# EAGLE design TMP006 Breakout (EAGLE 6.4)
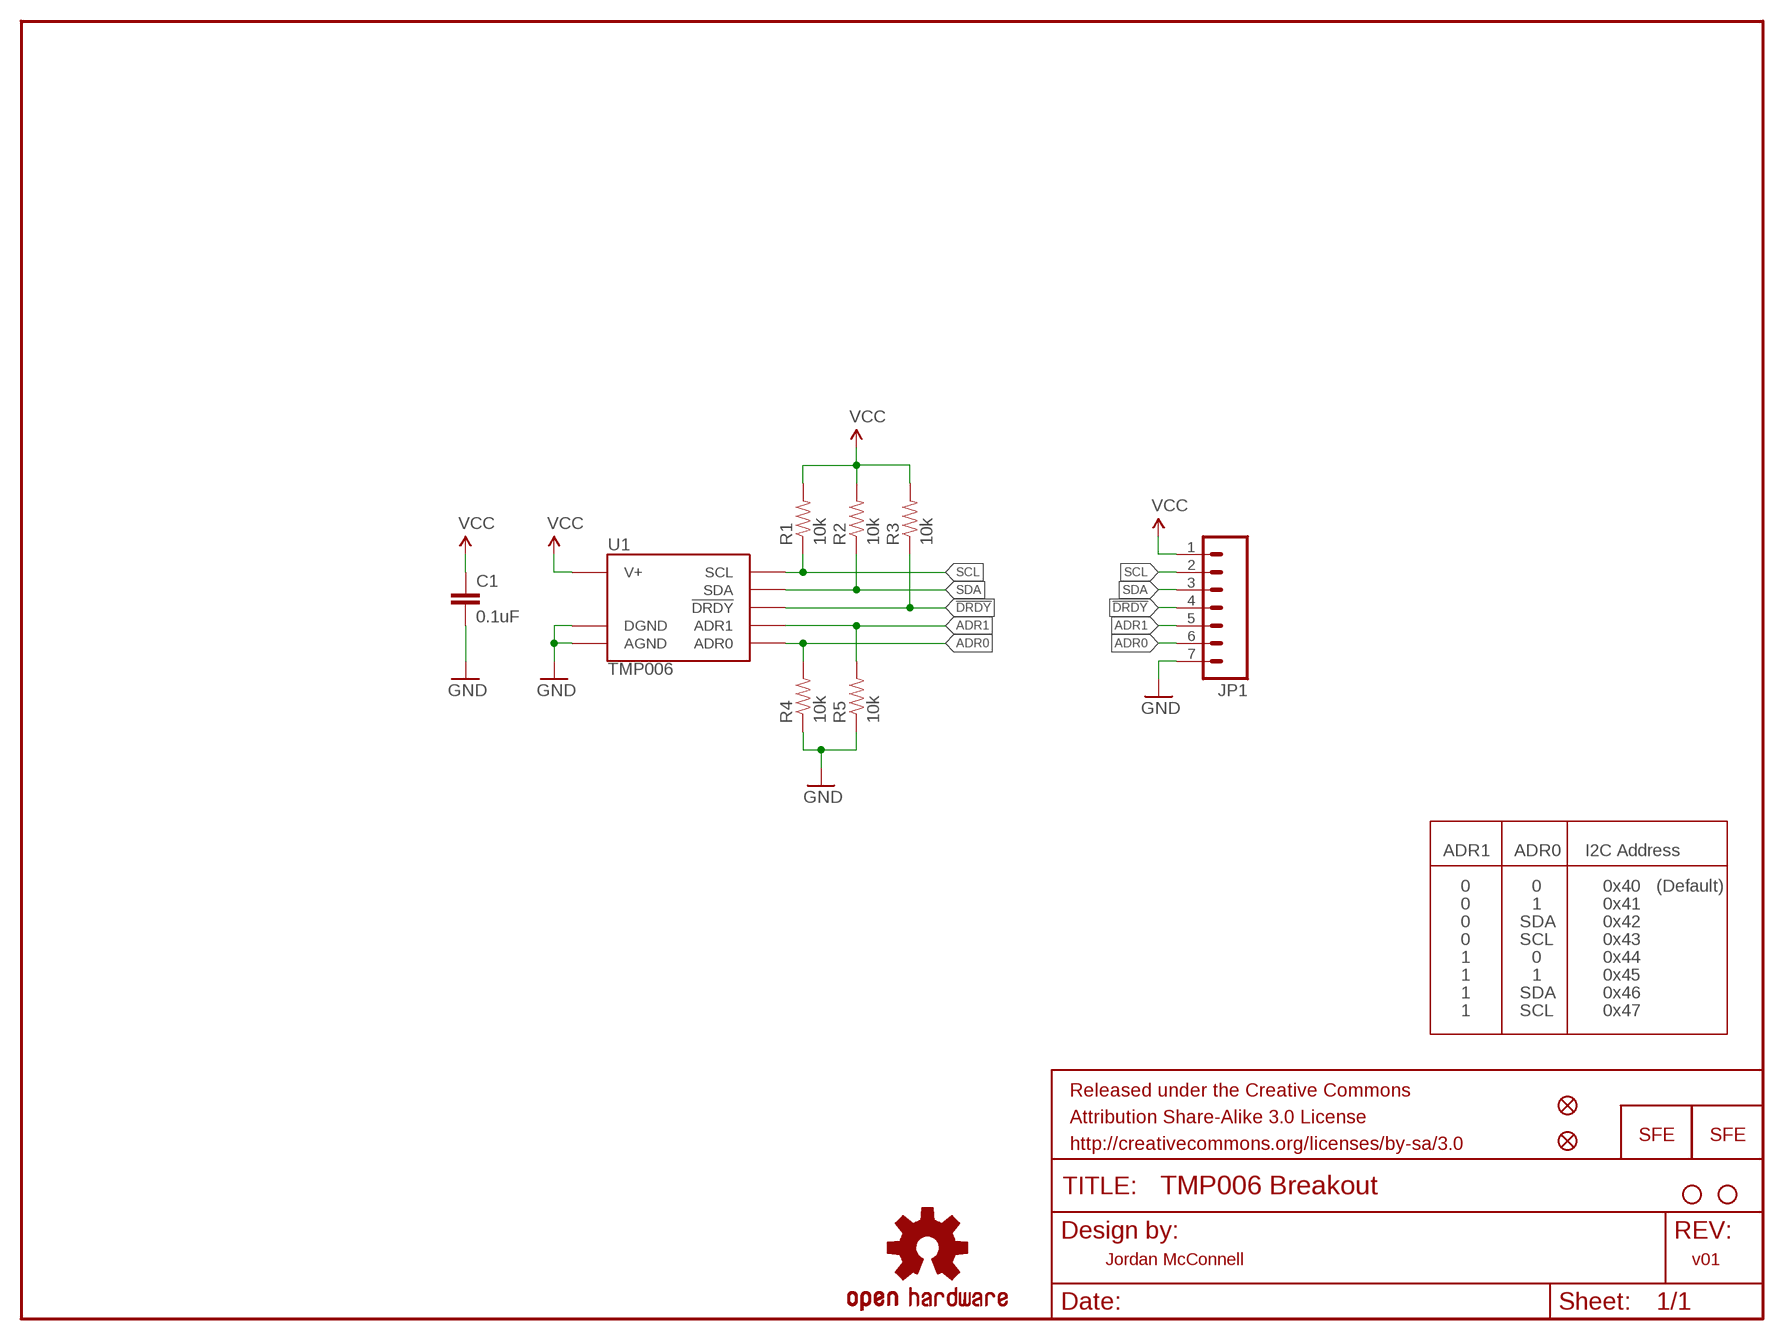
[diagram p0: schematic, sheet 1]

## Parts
C1  0.1uF  CAP0603-CAP  [0603-CAP]
FID1  FIDUCIALUFIDUCIAL  [MICRO-FIDUCIAL]
FID2  FIDUCIALUFIDUCIAL  [MICRO-FIDUCIAL]
FRAME1  FRAME-LETTER  [CREATIVE_COMMONS]
JP1  M07  [1X07]
LOGO1  LOGO-SFESK  [SFE-LOGO-FLAME]
LOGO2  OSHW-LOGOS  [OSHW-LOGO-S]
LOGO3  LOGO-SFENEW  [SFE-NEW-WEBLOGO]
R1  10k  RESISTOR0603-RES  [0603-RES]
R2  10k  RESISTOR0603-RES  [0603-RES]
R3  10k  RESISTOR0603-RES  [0603-RES]
R4  10k  RESISTOR0603-RES  [0603-RES]
R5  10k  RESISTOR0603-RES  [0603-RES]
STANDOFF1  STAND-OFF  [STAND-OFF]
STANDOFF2  STAND-OFF  [STAND-OFF]
U1  TMP006  [BGA8DS]

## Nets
!DRDY: JP1.4 R3.1 U1.C2(!DRDY)
ADR0: JP1.6 R4.2 U1.C1(ADR0)
ADR1: JP1.5 R5.2 U1.B1(ADR1)
GND: C1.2 JP1.7 R4.1 R5.1 U1.A1(DGND) U1.A2(AGND)
SCL: JP1.2 R1.1 U1.B3(SCL)
SDA: JP1.3 R2.1 U1.C3(SDA)
VCC: C1.1 JP1.1 R1.2 R2.2 R3.2 U1.A3(V+)

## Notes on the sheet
- ADR1 | ADR0 | I2C Address
- 0 | 0 | 0x40 | (Default)
- 0 | 1 | 0x41
- 0 | SDA | 0x42
- 0 | SCL | 0x43
- 1 | 0 | 0x44
- 1 | 1 | 0x45
- 1 | SDA | 0x46
- 1 | SCL | 0x47
- Jordan McConnell | v01

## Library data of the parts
C1 = SparkFun-Capacitors:CAP: Capacitor
FID1 FID2 = SparkFun-Aesthetics:FIDUCIAL: Fiducial Alignment Points
FRAME1 = SparkFun-Aesthetics:FRAME-LETTER: Schematic Frame
JP1 = SparkFun-Connectors:M07: Header 7 Standard 7-pin 0.1" header. Use with straight break away headers (SKU : PRT-00116), right angle break away headers (PRT-00553), swiss pins (PRT-00743), machine pins (PRT-00117), and female headers (PRT-00115). NOTES ON THE VARIANTS LOCK and LOCK_LONGPADS... This footprint was designed to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
LOGO1 LOGO3 = SparkFun-Aesthetics:LOGO-SFE: Spark Fun Electronics PCB Logo
LOGO2 = SparkFun-Aesthetics:OSHW-LOGO: Open Source Hardware Logo This logo indicates the piece of hardware it is found on incorporates a OSHW license and/or adheres to the definition of open source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
R1-R5 = SparkFun-Resistors:RESISTOR: Resistor
STANDOFF1 STANDOFF2 = SparkFun-Electromechanical:STAND-OFF: #4 Stand Off
U1 = SparkFun-DigitalIC:TMP006

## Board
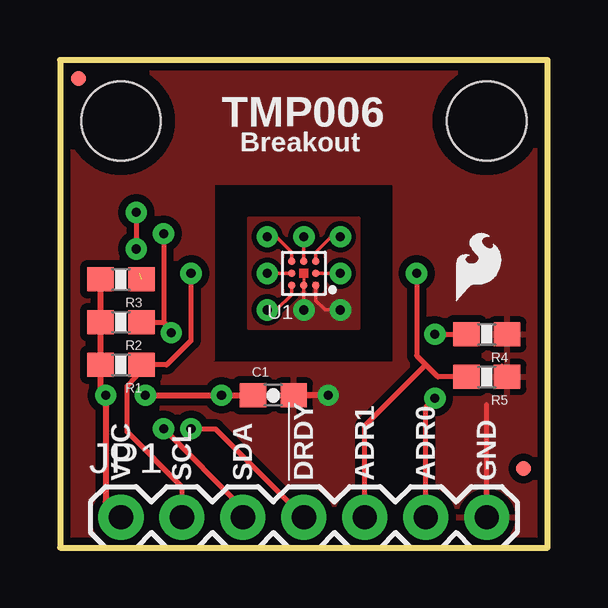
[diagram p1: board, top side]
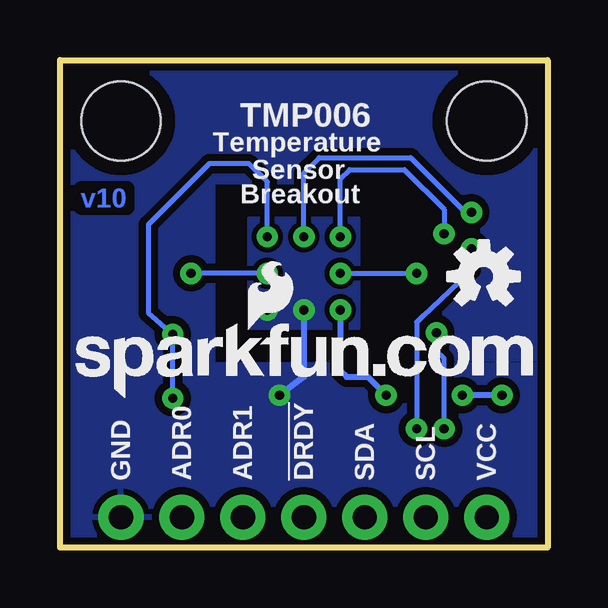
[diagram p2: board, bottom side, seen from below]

Size 20.32 x 20.32 mm. Coordinates in mm from the lower left corner, seen from the top.
Outline: 0,20.32 0,0 20.32,0 20.32,20.32 0,20.32
Copper layers (1*16): Top 0.035mm / dielectric 1.5mm / Bottom 0.035mm
Design rules "default": minimum track width 6mil, minimum drill 15mil, track to track 8mil, track to pad 8mil, pad to pad 8mil, via to via 8mil, smd to smd 8mil, copper to edge 8mil, drill to drill 8mil, minimum pad ring 12mil, minimum via ring 10mil, stop-mask expansion 4mil, vias tented up to drill 20mil, thermal gap 10mil
tRestrict: area 10.3,10.8 to 10.5,11; area 10.8,10.8 to 11,11

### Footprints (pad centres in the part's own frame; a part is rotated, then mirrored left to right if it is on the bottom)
0603-CAP = smd 1.1 x 1: 1 -0.85,0; 2 0.85,0
MICRO-FIDUCIAL = smd 0.635 x 0.635: 1 0,0
1X07 = drill 1.016 pad 1.88: 1 0,0; 2 2.54,0; 3 5.08,0; 4 7.62,0; 5 10.16,0; 6 12.7,0; 7 15.24,0
0603-RES = smd 1.1 x 1: 1 -0.85,0; 2 0.85,0
STAND-OFF = hole 3.302: 0,0
BGA8DS = smd 0.305 x 0.305: A1 0.5,-0.5; A2 0,-0.5; A3 -0.5,-0.5; B1 0.5,0; B3 -0.5,0; C1 0.5,0.5; C2 0,0.5; C3 -0.5,0.5

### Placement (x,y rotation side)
C1  8.89,6.35 0 top
FID1  19.3,3.3 0 top
FID2  0.76,19.56 0 top
FRAME1  not placed on the board
JP1  2.54,1.27 0 top
LOGO1  16.51,10.29 0 top
LOGO2  2.67,11.3 0 bottom
LOGO3  19.68,6.22 0 bottom
R1  2.54,7.62 180 top
R2  2.54,9.4 180 top
R3  2.54,11.18 180 top
R4  17.78,8.89 180 top
R5  17.78,7.11 180 top
STANDOFF1  2.54,17.78 0 top
STANDOFF2  17.78,17.78 0 top
U1  10.16,11.43 0 top

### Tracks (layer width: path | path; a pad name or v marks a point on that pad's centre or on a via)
!DRDY  (via drill 0.38)  (1 unrouted)
  Top 0.152: U1.C2 v10.16,12.95
  Top 0.203: v3.17,13.97 v3.17,12.45 | v5.46,4.95 6.48,4.95 JP1.4
  Bottom 0.203: v10.16,12.95 10.16,15.62 9.53,16.26 5.71,16.26 3.43,13.97 v3.17,13.97 | v5.46,4.95 5.46,9.4 5.21,9.65 3.3,11.43 3.17,11.56 v3.17,12.45
ADR0  (via drill 0.38)
  Top 0.152: U1.C1 10.66,12.31 11.3,12.95 v11.68,12.95
  Top 0.203: JP1.6 15.24,5.84 v15.62,6.22 | v15.62,8.89 R4.2
  Bottom 0.203: v11.68,12.95 11.68,15.24 12.45,16 14.1,16 16.64,13.46 16.64,13.08 16.64,9.78 v15.62,8.89 v15.62,6.22
ADR1  (via drill 0.38)
  Top 0.152: U1.B1 v11.68,11.43
  Top 0.203: v14.86,11.43 14.86,8 15.24,7.62 | JP1.5 12.7,5.08 15.24,7.62 | R5.2 15.75,7.11 15.24,7.62
  Bottom 0.203: v11.68,11.43 v14.86,11.43
GND  (via drill 0.38)
  Top 0.152: U1.A1 10.66,10.29 11.05,9.91 v11.68,9.91 | U1.A2 v10.16,9.91 | 18.41,7.61 R5.1
  Top 0.203: JP1.7 17.78,5.97 | 18.63,6.82 R5.1
  Top 0.254: v11.18,6.35 C1.2
  Bottom 0.254: v10.16,9.91 10.16,7.11 v11.18,6.35
  pour Top: 7.87,9.14 7.87,13.72 12.45,13.72 12.45,9.14
  pour Top (isolate 0.305): 0,7.62 0,0 20.32,0 20.32,20.32 0,20.32 0,7.87 6.35,7.87 6.35,15.24 13.97,15.24 13.97,7.62
  pour Bottom (isolate 0.305): 0,7.62 0,0 20.32,0 20.32,20.32 0,20.32 0,7.87 6.35,7.87 6.35,15.24 13.97,15.24 13.97,7.62
  pour Bottom: 7.87,13.72 12.45,13.72 12.45,9.14 7.87,9.14
SCL  (via drill 0.38)
  Top 0.152: U1.B3 v8.64,11.43 | 3.32,7.49 R1.1 3.17,7.61
  Top 0.203: JP1.2 5.08,2.54 2.79,4.83 2.79,6.73 3.17,7.11 3.17,7.61 | v5.46,11.43 5.46,8.64 4.45,7.62 R1.1
  Bottom 0.203: v8.64,11.43 v5.46,11.43
SDA  (via drill 0.38)
  Top 0.152: U1.C3 9.66,12.31 9.02,12.95 v8.64,12.95
  Top 0.203: JP1.3 7.62,1.65 v4.32,4.95 | v4.32,13.08 4.32,9.4 | 4.32,9.4 4.64,9.08 v4.64,8.95 | R2.1 4.32,9.4
  Bottom 0.203: v8.64,12.95 8.64,15.37 8.26,15.75 5.97,15.75 4.32,14.1 v4.32,13.08 | v4.32,4.95 4.32,7.87 4.64,8.19 v4.64,8.95
VCC  (via drill 0.38)
  Top 0.152: U1.A3 9.66,10.55 9.02,9.91 v8.64,9.91 | 1.91,7.61 R1.2
  Top 0.254: R3.2 R2.2 R1.2 1.69,6.57 v1.91,6.35 1.91,1.91 JP1.1 | v3.56,6.35 v6.73,6.35 C1.1
  Bottom 0.254: v8.64,9.91 8.64,7.37 8.38,7.11 7.49,7.11 v6.73,6.35 | v1.91,6.35 v3.56,6.35

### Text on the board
Bottom: v10
tPlace: TMP006 | Breakout | VCC | SCL | SDA | !DRDY | ADR1 | ADR0 | GND
bPlace: TMP006 | Temperature | Sensor | Breakout | VCC | SCL | SDA | !DRDY | ADR1 | ADR0 | GND
tValues: Jordan McConnell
